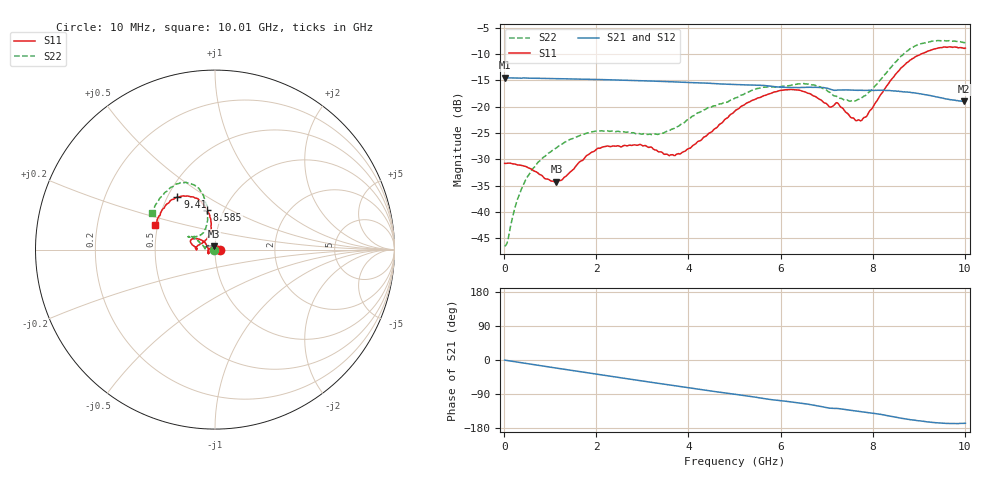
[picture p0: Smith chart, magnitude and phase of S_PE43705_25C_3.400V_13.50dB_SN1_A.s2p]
! Device ID: PE43705
! Serial: 1
! Insertion: A
! Impedance: 50 ohm
! Temp: 25C
! VDD: 3.400V
! Attenuation Step: 13.50dB
#  Hz  S  RI  R  50
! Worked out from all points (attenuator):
!   401 points, 10 MHz to 10.01 GHz, reference 50 ohm
!   highest |S21| = -14.50 dB at 10 MHz (marker M1); lowest = -19.0 dB at 9.985 GHz (marker M2)
!   lowest |S11| = -34.3 dB at 1.135 GHz (marker M3), VSWR 1.04, Z = 49.3 + j1.79 ohm
!   |S11| at or under -10 dB: start of sweep to 9.049 GHz
!   |S22| runs from -46.5 to -7.4 dB; largest |S21 - S12| = 0.0016
!   S11 on the Smith chart (normalised r, x): 10 MHz: 1.06, +0.00; 8.585 GHz: 0.83, +0.39; 9.41 GHz: 0.56, +0.38; 10.01 GHz: 0.49, +0.16
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1e7  0.029 0.000229  0.1883 -0.000799  0.1885 -0.000794  -0.00472 0.000462
8.5e7  0.029 0.00254  0.1877 -0.00563  0.1877 -0.00561  -0.0042 0.00351
2.85e8  0.0264 0.00953  0.1862 -0.018  0.1863 -0.0179  -0.00578 0.0117
4.6e8  0.0225 0.0154  0.1849 -0.0289  0.1849 -0.0286  -0.0088 0.0179
7.6e8  0.0105 0.0204  0.1801 -0.0464  0.1801 -0.0462  -0.0186 0.024
1.135e9  -0.00676 0.0182  0.1719 -0.0672  0.1719 -0.0671  -0.0331 0.0236
1.685e9  -0.0304 0.00442  0.1558 -0.0952  0.1558 -0.0952  -0.0522 0.0148
2.21e9  -0.04 -0.0131  0.1361 -0.1184  0.1362 -0.1184  -0.059 0.00322
2.935e9  -0.038 -0.0217  0.1035 -0.1436  0.1037 -0.1435  -0.0555 0.00308
3.36e9  -0.0332 -0.0171  0.0822 -0.1535  0.0824 -0.1533  -0.0546 0.00679
3.86e9  -0.0366 0.00316  0.0564 -0.1613  0.0566 -0.1611  -0.0658 0.0205
5.01e9  -0.0743 0.0529  -0.00149 -0.1625  -0.00127 -0.1625  -0.1062 0.0577
5.985e9  -0.1302 0.0579  -0.0454 -0.1466  -0.0447 -0.1467  -0.1354 0.0743
6.685e9  -0.1261 0.0265  -0.0727 -0.1342  -0.0727 -0.134  -0.1441 0.0716
7.335e9  -0.0947 0.0243  -0.0917 -0.1118  -0.0916 -0.112  -0.0909 0.0769
7.71e9  -0.0512 0.0542  -0.1023 -0.1003  -0.1019 -0.1003  -0.0612 0.1005
8.36e9  -0.0237 0.1692  -0.1206 -0.076  -0.1197 -0.0764  -0.0439 0.2238
8.585e9  -0.0442 0.2201  -0.124 -0.0635  -0.1233 -0.0645  -0.0598 0.2864
8.935e9  -0.096 0.2841  -0.1262 -0.0473  -0.1258 -0.0466  -0.1182 0.3614
9.41e9  -0.2099 0.2925  -0.1198 -0.0298  -0.1195 -0.0298  -0.2186 0.3645
9.985e9  -0.325 0.1485  -0.1095 -0.025  -0.1095 -0.0255  -0.3447 0.2136
1.001e10  -0.3321 0.1394  -0.1099 -0.0256  -0.1105 -0.0261  -0.3525 0.2028
